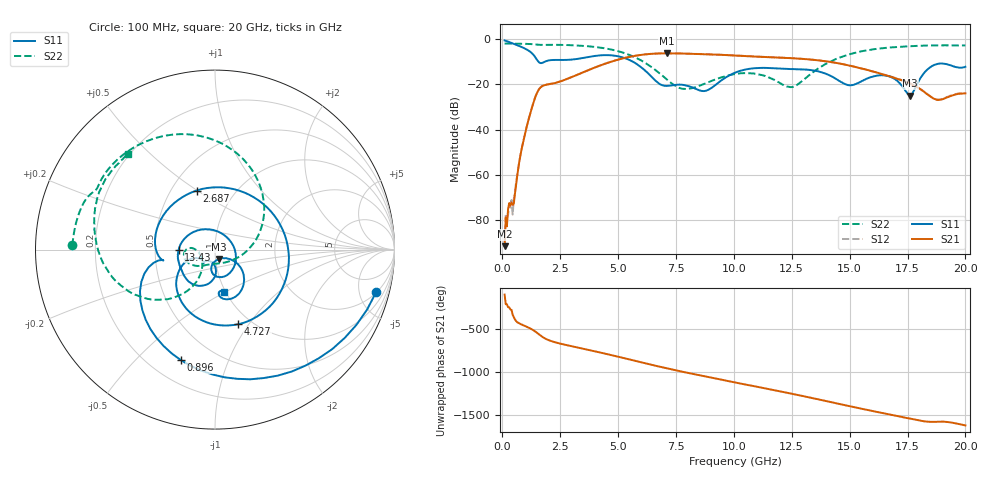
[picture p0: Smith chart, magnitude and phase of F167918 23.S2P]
!  2-Port S-parameters saved by WinCal
! VAR MeasName=S-Parameters (CALIBRATED_DATA) read from VNA (N5242A)
! VAR MeasDate=2016-11-22 10:25:51
! VAR NAME=F167918 23
! VAR FILENAME=F167918 23.S2P
! VAR DATE=2016-11-22 10:25:52
! VAR PHYS_PORTS=1,2
# Hz S DB R 50
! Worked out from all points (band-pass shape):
!   401 points, 100 MHz to 20 GHz, reference 50 ohm
!   highest |S21| = -6.32 dB at 7.115 GHz (marker M1); lowest = -91.5 dB at 100 MHz (marker M2)
!   |S21| within 3 dB of the highest: 4.93 GHz to 13.54 GHz (8.61 GHz wide, 93.2 % of centre)
!   lowest |S11| = -25.0 dB at 17.61 GHz (marker M3), VSWR 1.12, Z = 52 - j5.41 ohm
!   |S11| at or under -10 dB: 1.56 GHz to 1.841 GHz (281.6 MHz wide, 16.6 % of centre); 5.637 GHz to end of sweep
!   |S22| runs from -22.1 to -2.0 dB; largest |S21 - S12| = 0.0043
!   S11 on the Smith chart (normalised r, x): 100 MHz: 2.08, -7.12; 896 MHz: 0.33, -0.68; 2.687 GHz: 0.67, +0.50; 4.727 GHz: 0.87, -0.89; 13.43 GHz: 0.66, +0.00; 20 GHz: 0.98, -0.50
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1e8  -0.65 -14.8  -91.46 -94.0  -89.94 141.5  -2.00 178.3
4.4825e8  -1.91 -57.8  -73.15 29.1  -77.50 45.0  -2.04 172.5
8.96e8  -3.82 -107.3  -45.74 -92.2  -45.55 -91.8  -2.11 165.0
1.5925e9  -10.35 -169.0  -22.10 158.7  -22.05 158.6  -2.57 153.7
2.687e9  -9.26 107.2  -18.08 41.1  -18.07 40.8  -2.64 135.9
3.43325e9  -8.47 34.5  -14.95 -3.1  -14.96 -3.2  -2.99 119.9
4.03025e9  -7.44 -18.4  -12.44 -38.8  -12.44 -38.7  -3.54 104.8
4.72675e9  -7.22 -72.7  -9.94 -82.4  -9.90 -82.3  -4.70 84.1
5.62225e9  -9.92 -130.6  -7.64 -140.3  -7.59 -140.5  -7.59 51.5
6.7665e9  -19.64 -152.4  -6.38 145.4  -6.39 145.3  -14.95 -2.0
7.11475e9  -20.70 -137.1  -6.32 123.9  -6.33 123.9  -17.95 -22.9
8.7565e9  -22.93 -108.8  -6.70 29.8  -6.70 29.8  -19.66 -123.1
1.005e10  -14.88 -97.0  -7.28 -40.5  -7.27 -40.4  -15.47 -155.5
1.119425e10  -12.75 -126.7  -7.88 -101.2  -7.84 -101.0  -15.91 179.9
1.248775e10  -13.29 -152.8  -8.47 -171.1  -8.45 -171.3  -21.23 -153.0
1.338325e10  -13.83 -178.3  -9.13 137.7  -9.13 137.6  -14.94 -119.9
1.3433e10  -13.87 179.9  -9.22 134.9  -9.19 134.6  -14.52 -119.8
1.51245e10  -20.33 34.9  -12.03 35.2  -12.05 35.5  -6.36 -146.1
1.67165e10  -16.58 -87.6  -16.41 -53.9  -16.39 -53.3  -3.80 -178.4
1.7612e10  -24.96 -66.5  -19.68 -103.3  -19.56 -103.2  -3.21 166.6
1.8607e10  -11.69 -53.8  -26.20 -140.9  -26.06 -140.3  -2.83 150.9
2e10  -12.26 -78.0  -23.99 177.4  -23.81 177.7  -2.85 132.6
